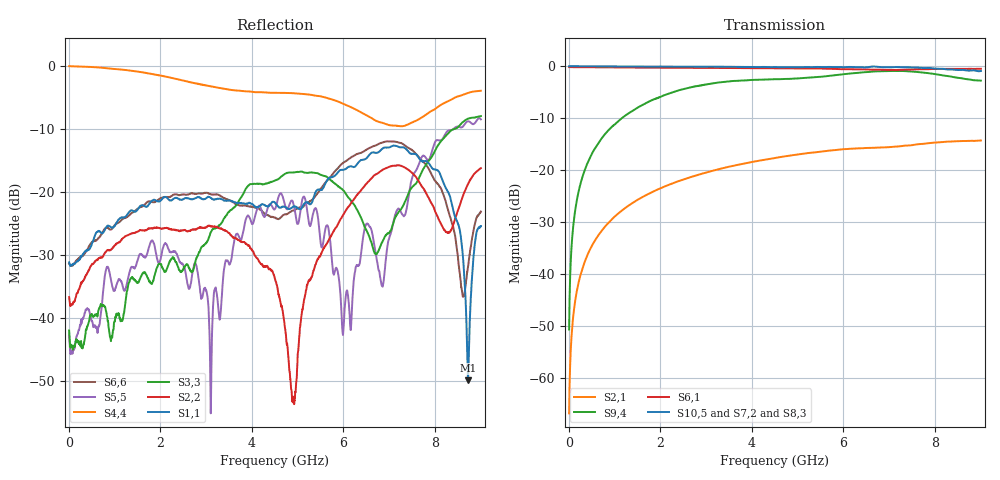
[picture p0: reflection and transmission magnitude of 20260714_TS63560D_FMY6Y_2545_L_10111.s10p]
# GHz S DB R 50
! CMT, SN0916, 25263762, 26.7.0
! Date: 15.07.2026 13:46:10
! Data: Format
! Freq S1.1:dB/Ang S1.2:dB/Ang S1.3:dB/Ang S1.4:dB/Ang S1.5:dB/Ang S1.6:dB/Ang S1.7:dB/Ang S1.8:dB/Ang S1.9:dB/Ang S1.10:dB/Ang
!  S2.1:dB/Ang S2.2:dB/Ang S2.3:dB/Ang S2.4:dB/Ang S2.5:dB/Ang S2.6:dB/Ang S2.7:dB/Ang S2.8:dB/Ang S2.9:dB/Ang S2.10:dB/Ang
!  S3.1:dB/Ang S3.2:dB/Ang S3.3:dB/Ang S3.4:dB/Ang S3.5:dB/Ang S3.6:dB/Ang S3.7:dB/Ang S3.8:dB/Ang S3.9:dB/Ang S3.10:dB/Ang
!  S4.1:dB/Ang S4.2:dB/Ang S4.3:dB/Ang S4.4:dB/Ang S4.5:dB/Ang S4.6:dB/Ang S4.7:dB/Ang S4.8:dB/Ang S4.9:dB/Ang S4.10:dB/Ang
!  S5.1:dB/Ang S5.2:dB/Ang S5.3:dB/Ang S5.4:dB/Ang S5.5:dB/Ang S5.6:dB/Ang S5.7:dB/Ang S5.8:dB/Ang S5.9:dB/Ang S5.10:dB/Ang
!  S6.1:dB/Ang S6.2:dB/Ang S6.3:dB/Ang S6.4:dB/Ang S6.5:dB/Ang S6.6:dB/Ang S6.7:dB/Ang S6.8:dB/Ang S6.9:dB/Ang S6.10:dB/Ang
!  S7.1:dB/Ang S7.2:dB/Ang S7.3:dB/Ang S7.4:dB/Ang S7.5:dB/Ang S7.6:dB/Ang S7.7:dB/Ang S7.8:dB/Ang S7.9:dB/Ang S7.10:dB/Ang
!  S8.1:dB/Ang S8.2:dB/Ang S8.3:dB/Ang S8.4:dB/Ang S8.5:dB/Ang S8.6:dB/Ang S8.7:dB/Ang S8.8:dB/Ang S8.9:dB/Ang S8.10:dB/Ang
!  S9.1:dB/Ang S9.2:dB/Ang S9.3:dB/Ang S9.4:dB/Ang S9.5:dB/Ang S9.6:dB/Ang S9.7:dB/Ang S9.8:dB/Ang S9.9:dB/Ang S9.10:dB/Ang
!  S10.1:dB/Ang S10.2:dB/Ang S10.3:dB/Ang S10.4:dB/Ang S10.5:dB/Ang S10.6:dB/Ang S10.7:dB/Ang S10.8:dB/Ang S10.9:dB/Ang S10.10:dB/Ang
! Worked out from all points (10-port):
!   2001 points, 10 MHz to 9 GHz, reference 50 ohm
!   strongest paths, dB at 10 MHz, 2.257 GHz, 4.505 GHz, 6.753 GHz, 9 GHz:
!     S10,5: -0.1, -0.2, -0.2, -0.2, -1.0
!     S7,2: -0.1, -0.3, -0.4, -0.6, -0.6
!     S8,3: -0.1, -0.2, -0.4, -0.4, -1.2
!     S6,1: -0.3, -0.4, -0.5, -0.7, -0.6
!     S9,4: -50.8, -5.1, -2.6, -1.1, -2.9
!     S2,1: -66.9, -22.7, -17.7, -15.7, -14.4
!   lowest |S11| = -49.8 dB at 8.721 GHz (marker M1), VSWR 1.01, Z = 49.9 + j0.292 ohm
!   |S11| at or under -10 dB: start of sweep to end of sweep
